FUNCTION FC 65 : VOID
TITLE =BLOCK MOVING BOLSTER PUMP
AUTHOR : Esposito
FAMILY : EGAL_srl
NAME : MOV_BOLS
VERSION : 0.1

BEGIN
NETWORK
TITLE =CONDITIONS FOR START MOVING BOLSTER
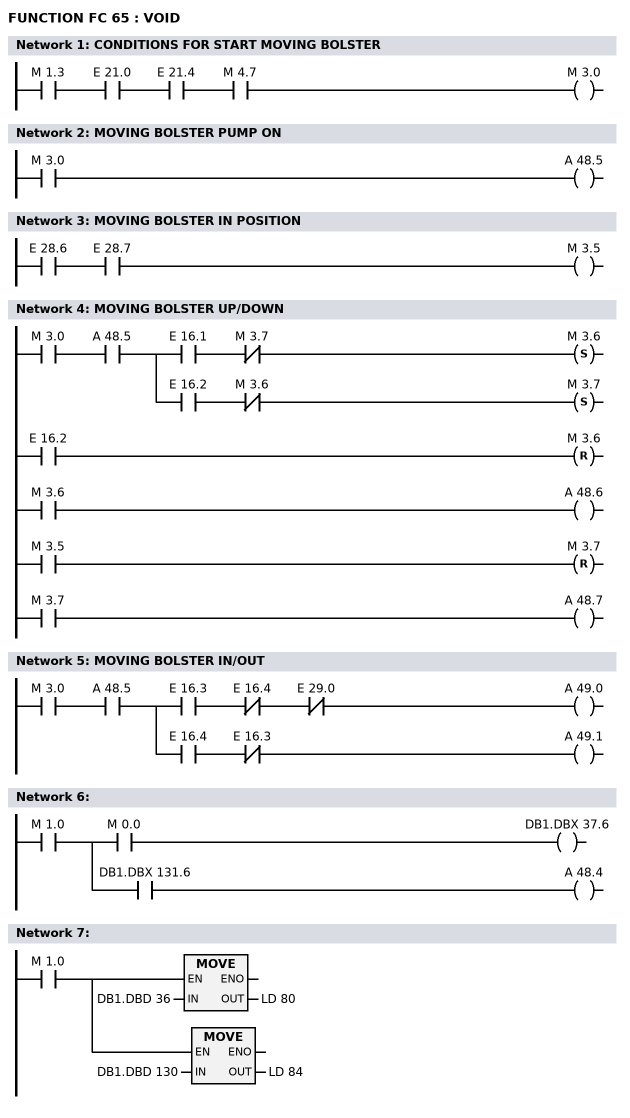
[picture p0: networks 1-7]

      U     M      1.3;
      U     E     21.0;
      U     E     21.4;
      U     M      4.7;
      =     M      3.0;
NETWORK
TITLE =MOVING BOLSTER PUMP ON

      U     M      3.0;
      =     A     48.5;
NETWORK
TITLE =MOVING BOLSTER IN POSITION

      U     E     28.6;
      U     E     28.7;
      =     M      3.5;
NETWORK
TITLE =MOVING BOLSTER UP/DOWN

      U     M      3.0;
      U     A     48.5;
      =     L     88.0;
      U     L     88.0;
      U     E     16.1;
      UN    M      3.7;
      S     M      3.6;
      U     E     16.2;
      R     M      3.6;
      U     M      3.6;
      =     A     48.6;
      U     L     88.0;
      U     E     16.2;
      UN    M      3.6;
      S     M      3.7;
      U     M      3.5;
      R     M      3.7;
      U     M      3.7;
      =     A     48.7;
NETWORK
TITLE =MOVING BOLSTER IN/OUT

      U     M      3.0;
      U     A     48.5;
      =     L     88.0;
      U     L     88.0;
      U     E     16.3;
      UN    E     16.4;
      UN    E     29.0;
      =     A     49.0;
      U     L     88.0;
      U     E     16.4;
      UN    E     16.3;
      =     A     49.1;
NETWORK
TITLE =

      U     M      1.0;
      =     L     88.0;
      U     L     88.0;
      U     M      0.0;
      =     DB1.DBX   37.6;
      U     L     88.0;
      U     DB1.DBX  131.6;
      =     A     48.4;
NETWORK
TITLE =

      U     M      1.0;
      =     L     88.0;
      U     L     88.0;
      SPBNB M001;
      L     DB1.DBD   36;
      T     LD    80;
M001: NOP   0;
      U     L     88.0;
      SPBNB M002;
      L     DB1.DBD  130;
      T     LD    84;
M002: NOP   0;
END_FUNCTION

